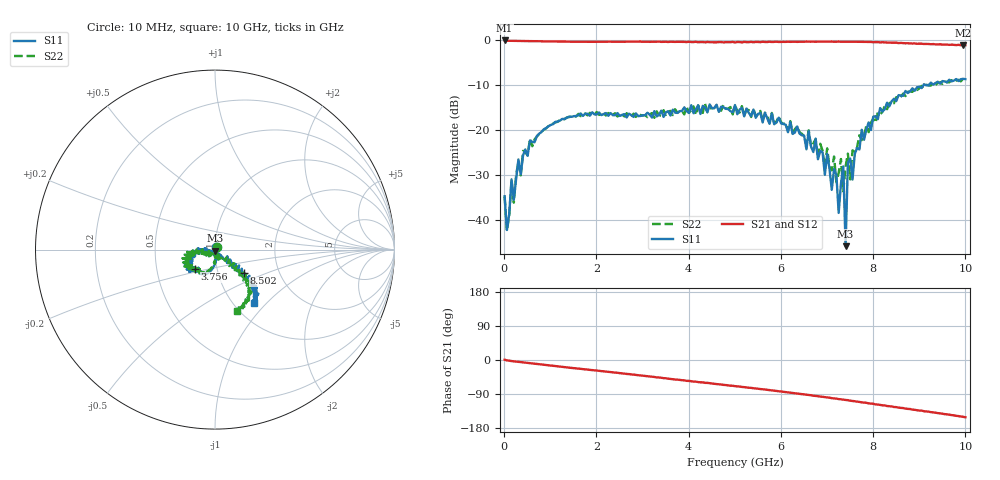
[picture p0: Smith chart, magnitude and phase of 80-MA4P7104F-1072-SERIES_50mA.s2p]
!Agilent Technologies,E8364C,MY48140145,A.09.42.15
!Agilent E8364C: A.09.42.15
!Date: Wednesday, December 02, 2020 07:35:27
!Correction: S11(Full 2 Port(1,2))
!S21(Full 2 Port(1,2))
!S12(Full 2 Port(1,2))
!S22(Full 2 Port(1,2))
!S2P File: Measurements: S11, S21, S12, S22:
# Hz S  dB  R 50
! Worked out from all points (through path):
!   201 points, 10 MHz to 10 GHz, reference 50 ohm
!   highest |S21| = -0.06 dB at 10 MHz (marker M1); lowest = -1.1 dB at 9.95 GHz (marker M2)
!   group delay of S21, straight-line fit = 41 ps
!   lowest |S11| = -45.9 dB at 7.403 GHz (marker M3), VSWR 1.01, Z = 50 - j0.507 ohm
!   |S11| at or under -10 dB: start of sweep to 9.091 GHz; 9.139 GHz to 9.207 GHz (68.08 MHz wide, 0.742 % of centre)
!   |S22| runs from -42.5 to -8.6 dB; largest |S21 - S12| = 0.015
!   S11 on the Smith chart (normalised r, x): 10 MHz: 1.02, +0.03; 3.756 GHz: 0.78, -0.17; 8.502 GHz: 1.33, -0.37; 10 GHz: 1.23, -0.85
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1e7  -34.77 63.7  -0.06 0.8  -0.02 -0.1  -34.84 43.6
5.995e7  -42.29 -47.9  -0.13 -1.0  -0.12 -1.1  -42.50 -60.5
1.5985e8  -31.01 -72.9  -0.14 -2.8  -0.14 -2.7  -31.28 -73.0
2.098e8  -35.54 -64.8  -0.14 -3.5  -0.14 -3.5  -36.22 -75.0
5.5945e8  -22.35 -91.2  -0.23 -8.6  -0.23 -8.6  -21.94 -90.7
1.7083e9  -16.88 -114.5  -0.35 -24.1  -0.33 -23.9  -16.63 -119.8
3.35665e9  -16.62 -134.9  -0.32 -46.2  -0.34 -46.4  -16.72 -128.7
3.75625e9  -16.21 -135.6  -0.37 -51.8  -0.41 -52.0  -16.17 -133.1
5.005e9  -14.45 -152.2  -0.51 -69.0  -0.47 -68.8  -14.52 -165.1
6.7033e9  -24.93 179.8  -0.32 -94.2  -0.30 -93.8  -22.98 177.9
7.15285e9  -28.70 -176.9  -0.35 -101.3  -0.34 -101.7  -25.92 -132.3
7.25275e9  -38.48 -165.0  -0.31 -103.2  -0.33 -102.8  -29.53 -151.2
7.35265e9  -28.11 -61.7  -0.35 -104.7  -0.31 -104.4  -33.67 -64.8
7.4026e9  -45.89 -89.0  -0.34 -105.5  -0.33 -105.6  -28.11 -104.9
7.45255e9  -27.30 -72.3  -0.35 -106.0  -0.34 -106.4  -25.28 -61.8
7.5025e9  -26.36 -44.7  -0.35 -107.4  -0.32 -107.0  -31.03 -52.7
7.55245e9  -31.06 -49.5  -0.35 -108.1  -0.36 -108.3  -24.54 -72.5
7.7023e9  -24.36 -47.7  -0.36 -110.5  -0.39 -110.8  -21.18 -51.9
8.35165e9  -14.75 -35.4  -0.52 -122.0  -0.54 -122.1  -14.08 -46.5
8.5015e9  -13.57 -39.1  -0.57 -124.4  -0.60 -124.8  -12.70 -45.2
9.95005e9  -8.62 -51.3  -1.13 -150.1  -1.15 -150.0  -8.60 -70.2
1e10  -8.67 -54.2  -1.12 -151.0  -1.12 -151.1  -8.79 -69.9
